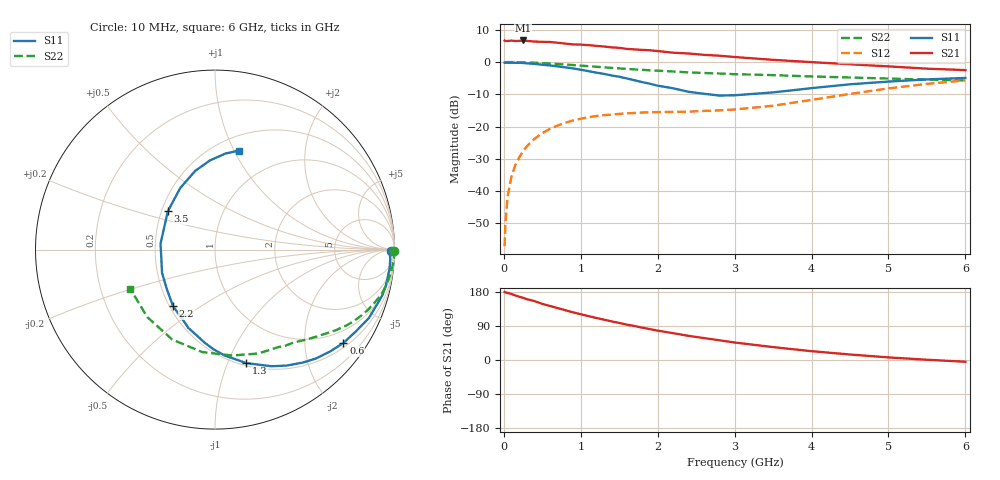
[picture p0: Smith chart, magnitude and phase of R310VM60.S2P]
! SIEMENS Small Signal Semiconductors
! BFR181
! Si NPN RF Bipolar Junction Transistor in SOT23
! VCE = 10 V  IC = 0.6 mA
! Common Emitter S-Parameters:  May  1996
# GHz  S  MA  R  50
!  f  S11  S21  S12  S22
! GHz  MAG  ANG  MAG  ANG  MAG  ANG  MAG  ANG
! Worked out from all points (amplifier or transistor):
!   36 points, 10 MHz to 6 GHz, reference 50 ohm
!   highest |S21| = 6.7 dB at 250 MHz (marker M1)
!   |S21| within 3 dB of that: start of sweep to 1.86 GHz
!   unconditionally stable (mu >= 1): 2.334 GHz to 3.944 GHz
!   at 250 MHz: K = 0.13, MSG = 17.2 dB, |S12| = -27.6 dB
!   at 1.4 GHz: K = 0.63, MSG = 10.4 dB, |S12| = -16.3 dB
!   at 6 GHz: K = 0.90, MSG = 1.6 dB, |S12| = -5.7 dB
!   S11 on the Smith chart (normalised r, x): 10 MHz: 81, -45; 600 MHz: 0.62, -2.96; 1.3 GHz: 0.53, -1.17; 2.2 GHz: 0.52, -0.39; 3.5 GHz: 0.54, +0.26; 6 GHz: 0.64, +1.04
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0.01  0.9812 -0.6  2.15 179.5  0.0014 89.1  0.9994 -0.3
0.02  0.9744 -1.2  2.12 178.5  0.0032 88.1  0.9935 -0.6
0.05  0.9782 -3.1  2.121 177.1  0.0084 86.5  0.9981 -1.4
0.1  0.9785 -6.2  2.149 174.1  0.017 85.9  0.998 -2.9
0.15  0.9744 -9.0  2.117 170.1  0.0255 84.3  0.9949 -4.5
0.25  0.9666 -15.2  2.16 163.9  0.0416 79.1  0.9889 -7.4
0.4  0.9383 -24.0  2.074 155.3  0.0648 73.2  0.9754 -11.5
0.5  0.9077 -30.1  2.057 148.1  0.079 69.5  0.9633 -14.3
0.6  0.8848 -36.0  2.043 142.6  0.0923 65.9  0.947 -16.9
0.8  0.8265 -47.3  1.93 131.3  0.1145 58.6  0.914 -21.7
1.1  0.7225 -64.1  1.83 115.9  0.1395 50.3  0.8629 -28.0
1.3  0.6558 -74.6  1.741 106.6  0.1502 45.8  0.8276 -31.7
1.6  0.5558 -90.8  1.597 93.2  0.1604 40.8  0.783 -36.3
1.8  0.4879 -102.2  1.543 85.3  0.165 39.0  0.7569 -39.1
2.2  0.3922 -126.7  1.396 70.8  0.1687 37.4  0.7131 -44.8
2.4  0.3458 -141.2  1.357 63.8  0.1702 38.3  0.692 -47.5
2.8  0.3024 -171.6  1.253 52.1  0.1782 41.0  0.6645 -53.5
3.5  0.3386 140.9  1.082 34.0  0.2103 47.9  0.627 -67.4
4.5  0.4519 104.2  0.923 14.5  0.3206 49.3  0.5753 -97.1
5  0.4978 93.2  0.856 6.8  0.3901 44.7  0.5549 -115.4
5.5  0.5383 83.8  0.79 0.7  0.4584 37.6  0.5328 -135.0
6  0.5664 76.6  0.75 -4.6  0.5199 29.3  0.5202 -155.1
